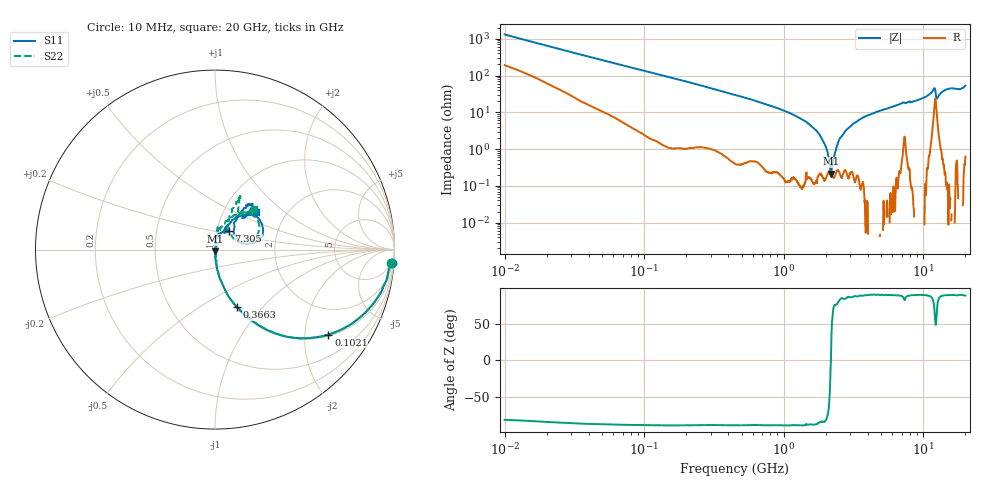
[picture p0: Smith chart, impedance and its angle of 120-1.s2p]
!Keysight Technologies,P5008B,MY61100088,A.16.20.02
!Date: Monday, May 27, 2024 17:10:48
!Correction: S11(C* 2-Port  )
!S21(C* 2-Port  )
!S12(C* 2-Port  )
!S22(C* 2-Port  )
!S2P File: Measurements: S11, S21, S12, S22:Log Frequency Sweep
# Hz S  dB  R 50
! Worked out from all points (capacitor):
!   1601 points, 10 MHz to 20 GHz, reference 50 ohm
!   read as one part in series: C = 12.3 pF near 10.39 MHz
!   lowest |Z| = 215 mohm at 2.175 GHz (marker M1)
!   series resonance near 2.176 GHz, so ESL is about 430 pH
!   S11 on the Smith chart (normalised r, x): 10 MHz: 4, -26; 102.1 MHz: 1.05, -2.64; 366.3 MHz: 1.01, -0.73; 7.305 GHz: 1.14, +0.24; 20 GHz: 1.41, +0.66
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1e7  -0.10 -4.3  -22.46 77.3  -22.47 77.4  -0.13 -4.3
3.555162e7  -0.42 -15.0  -11.71 72.0  -11.72 72.0  -0.43 -15.0
1.020651e8  -2.05 -36.8  -4.45 52.2  -4.46 52.2  -2.04 -36.9
1.263918e8  -2.78 -42.6  -3.40 46.6  -3.41 46.6  -2.77 -42.7
3.66322e8  -9.31 -69.0  -0.60 19.8  -0.61 19.9  -9.31 -69.1
4.472136e8  -10.88 -73.0  -0.41 16.4  -0.42 16.4  -10.87 -73.0
9.206888e8  -17.75 -82.3  -0.09 6.9  -0.10 6.9  -17.77 -82.0
1.589917e9  -26.51 -87.5  -0.01 1.9  -0.02 1.9  -26.26 -83.4
2.016191e9  -33.70 -87.8  0.00 -0.0  -0.01 -0.0  -32.83 -75.6
2.175414e9  -39.53 -81.4  0.00 -0.6  -0.01 -0.6  -37.29 -62.6
2.403631e9  -49.43 -17.3  0.01 -1.5  -0.00 -1.5  -42.25 -17.4
2.556753e9  -42.75 74.9  0.00 -2.0  -0.00 -2.0  -41.54 44.5
2.798263e9  -35.25 78.7  0.01 -2.8  -0.00 -2.8  -34.52 63.5
3.151135e9  -30.80 85.1  0.01 -3.8  -0.01 -3.9  -29.75 73.2
3.846973e9  -26.22 92.2  0.00 -5.9  -0.01 -5.9  -25.09 74.6
5.652411e9  -21.36 78.3  -0.01 -10.2  -0.02 -10.2  -21.40 80.4
7.305392e9  -17.82 53.7  -0.20 -14.1  -0.21 -14.1  -18.88 74.8
9.30816e9  -18.42 63.5  -0.02 -18.6  -0.03 -18.6  -18.30 77.5
1.174784e10  -11.45 46.2  -0.70 -28.6  -0.71 -28.6  -11.69 53.1
1.27966e10  -15.80 48.0  -0.32 -21.7  -0.33 -21.7  -16.25 61.5
1.511139e10  -9.99 53.0  -0.40 -30.6  -0.41 -30.6  -9.95 64.1
2e10  -10.14 42.9  -0.42 -43.3  -0.43 -43.3  -10.08 46.5
